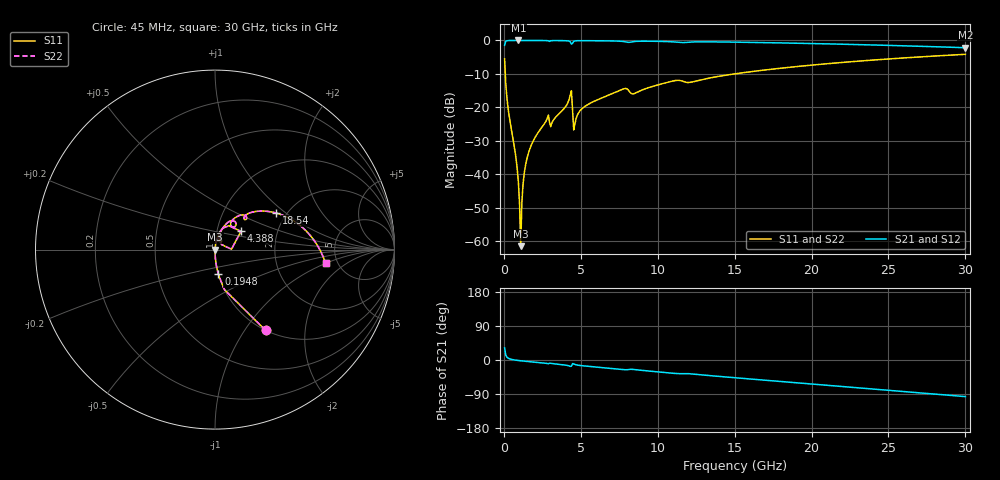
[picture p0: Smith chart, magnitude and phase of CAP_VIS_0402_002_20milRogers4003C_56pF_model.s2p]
! S-parameter model data by Modelithics Inc.  support@modelithics.com  813-866-6335  Tampa FL USA
! S-Parameter data specifications:
! Substrate: 20-mil Rogers 4003C, substrate thickness, H=0.508mm, Dielectric constant, Er=3.75
! PCB Mounting Pad Footprint: Pad width, PadW=0.50mm , Pad length, PadL=0.50mm , Pad gap, PadG (edge-to-edge)=0.40mm , Reference planes=1.4mm apart
! Created Wed Nov 18 12:56:02 2015
# hz S ma R 50
! 2 Port Network Data from SP1.SP block
! freq  magS11  angS11  magS21  angS21  magS12  angS12  magS22  angS22
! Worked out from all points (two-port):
!   401 points, 45 MHz to 30 GHz, reference 50 ohm
!   highest |S21| = -0.01 dB at 943.6 MHz (marker M1); lowest = -2.2 dB at 30 GHz (marker M2)
!   |S21| within 3 dB of the highest: start of sweep to end of sweep
!   lowest |S11| = -61.5 dB at 1.093 GHz (marker M3), VSWR 1.00, Z = 50.1 + j0.0261 ohm
!   |S11| at or under -10 dB: 90.77 MHz to 14.99 GHz (14.9 GHz wide, 198 % of centre)
!   |S22| runs from -61.5 to -4.1 dB; largest |S21 - S12| = 0
!   S11 on the Smith chart (normalised r, x): 45 MHz: 1.00, -1.26; 194.8 MHz: 1.00, -0.28; 4.388 GHz: 1.31, +0.27; 18.54 GHz: 1.77, +0.85; 30 GHz: 4.01, -0.99
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4.5e7  0.5319 -57.9  0.8466 32.0  0.8466 32.0  0.5319 -57.9
1.94775e8  0.1393 -82.2  0.9899 7.6  0.9899 7.6  0.1393 -82.2
7.93875e8  0.01671 -88.2  0.9992 -0.5  0.9992 -0.5  0.01671 -88.2
9.4365e8  0.007476 -85.7  0.9992 -1.4  0.9992 -1.4  0.007476 -85.7
1.093425e9  0.0008448 18.0  0.9992 -2.1  0.9992 -2.1  0.0008448 18.0
1.2432e9  0.0071 80.4  0.9991 -2.7  0.9991 -2.7  0.0071 80.4
1.318088e9  0.01021 82.0  0.999 -3.1  0.999 -3.1  0.01021 82.0
1.467862e9  0.01607 83.0  0.9989 -3.7  0.9989 -3.7  0.01607 83.0
1.917188e9  0.0319 82.6  0.9984 -5.4  0.9984 -5.4  0.0319 82.6
2.74095e9  0.06259 78.8  0.9953 -8.8  0.9953 -8.8  0.06259 78.8
4.2387e9  0.1318 67.8  0.976 -15.5  0.976 -15.5  0.1318 67.8
4.388475e9  0.177 35.1  0.8796 -16.2  0.8796 -16.2  0.177 35.1
4.688025e9  0.06758 69.7  0.9886 -12.7  0.9886 -12.7  0.06758 69.7
5.062462e9  0.09484 73.1  0.9921 -15.0  0.9921 -15.0  0.09484 73.1
7.758412e9  0.1882 58.9  0.9635 -25.4  0.9635 -25.4  0.1882 58.9
8.4324e9  0.1597 55.5  0.9608 -24.9  0.9608 -24.9  0.1597 55.5
1.007992e10  0.2189 56.6  0.9688 -31.6  0.9688 -31.6  0.2189 56.6
1.50225e10  0.317 42.3  0.943 -46.8  0.943 -46.8  0.317 42.3
1.854221e10  0.3966 30.9  0.9133 -58.5  0.9133 -58.5  0.3966 30.9
2.003996e10  0.4286 26.1  0.8988 -63.4  0.8988 -63.4  0.4286 26.1
2.505742e10  0.5299 9.6  0.8429 -80.0  0.8429 -80.0  0.5299 9.6
3e10  0.6205 -7.0  0.7784 -96.6  0.7784 -96.6  0.6205 -7.0
